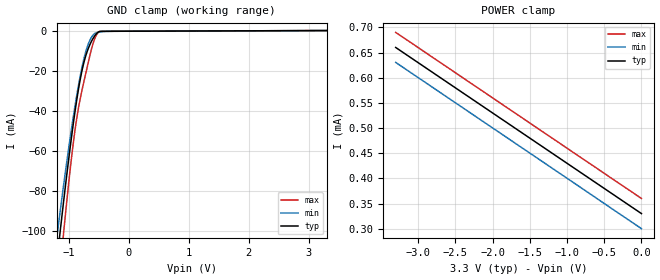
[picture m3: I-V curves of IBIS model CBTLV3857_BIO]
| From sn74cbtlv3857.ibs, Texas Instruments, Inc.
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[Model]   CBTLV3857_BIO
Model_type  Terminator
| variable   typ   min   max
C_comp   3.12pF   2.59pF   3.57pF
| C_tri-state   3.12pF   2.59pF   3.57pF
[Temperature Range]   40   100   -40
| Ambient temperature   25   85   -40
[Voltage range]   3.3   3   3.6
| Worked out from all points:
|   GND clamp passes 1 mA (typ) near -0.53 V on its own axis
[GND Clamp]
| CBTLV3857_BIO
|   Voltage   I(typ)   I(min)   I(max)
-3.3V     -769.1mA   -675.4mA   -909.9mA
-1.19V    -113.7mA   -101.9mA   -134.7mA
-1.135V   -98.92mA   -89.02mA   -117.2mA
-1.085V   -85.82mA   -77.59mA   -101.6mA
-920mV    -46.06mA   -42.63mA   -55.7mA
-860mV    -33.72mA   -31.45mA   -42.87mA
-800mV    -23.24mA   -21.53mA   -32.9mA
-735mV    -14.56mA   -12.67mA   -23.95mA
-670mV    -8.521mA   -6.271mA   -15.41mA
-545mV    -1.573mA   -824.4uA   -2.417mA
-440mV    -62.4uA    -197.5uA   -49.93uA
3.3V      330uA      330.1uA    330uA
[POWER Clamp]
| CBTLV3857_BIO
|   Voltage   I(typ)   I(min)   I(max)
-3.3V     660uA      630.4uA    690uA
-775mV    407.5uA    377.7uA    437.5uA
-475mV    377.5uA    347.6uA    407.5uA
-48.03fV  330uA      300.1uA    360uA
